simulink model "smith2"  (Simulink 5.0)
settings: Solver=ode45  StartTime=0.0  StopTime=100.0  FixedStep=0.1  RelTol=1e-3
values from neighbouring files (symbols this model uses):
  D = uicontrol(gcf,   'Style','edit',   'ForegroundColor','black',   'BackgroundColor',[1 1 1],   'String',num2str(D),   'Position',[100 18 80 20],   'CallBack',['D=str2num(get(D,''String''));'])    [sus1.m]    (also in sus2.m = uicontrol(gcf,   'Style','edit',   'ForegroundColor','black')
  p0 = P(3,1)    [simulacia11.m]    (also in simulacia12.m = P(1,4); simulacia21.m = P(1,4); simulacia22.m = P(1,5); smith.m = P(2,1))
  p1 = P(2,1)    [simulacia11.m]    (also in simulacia12.m = P(1,3); simulacia21.m = P(1,3); simulacia22.m = P(1,4); smith.m = P(1,1))
  p2 = P(1,1)    [simulacia11.m]    (also in simulacia12.m = P(1,2); simulacia21.m = P(1,2); simulacia22.m = P(1,3); smith.m = 0)
  p3 = 0    [simulacia11.m]    (also in simulacia12.m = P(1,1); simulacia21.m = P(1,1); simulacia22.m = P(1,2); smith.m)
  p4 = 0    [simulacia21.m]    (also in simulacia22.m = P(1,1); smithd.m)
  q0 = P(6,1)    [simulacia11.m]    (also in simulacia12.m = Q(1,4); simulacia21.m = Q(1,4); simulacia22.m = Q(1,5); smith.m = P(4,1))
  q1 = P(5,1)    [simulacia11.m]    (also in simulacia12.m = Q(1,3); simulacia21.m = Q(1,3); simulacia22.m = Q(1,4); smith.m = P(3,1))
  q2 = P(4,1)    [simulacia11.m]    (also in simulacia12.m = Q(1,2); simulacia21.m = Q(1,2); simulacia22.m = Q(1,3); smith.m = 0)
  q3 = 0    [simulacia11.m]    (also in simulacia12.m = Q(1,1); simulacia21.m = Q(1,1); simulacia22.m = Q(1,2); smith.m)
  q4 = 0    [simulacia21.m]    (also in simulacia22.m = Q(1,1); smithd.m)
  T = uicontrol(gcf,   'Style','edit',   'ForegroundColor','black',   'BackgroundColor',[1 1 1],   'String',num2str(T),   'Position',[100 40 80 20],   'CallBack',['T=str2num(get(T,''String''));'])    [sus1.m]    (also in sus2.m = uicontrol(gcf,   'Style','edit',   'ForegroundColor','black')
  Xi = uicontrol(gcf,   'Style','edit',   'ForegroundColor','black',   'BackgroundColor',[1 1 1],   'String',num2str(Xi),   'Position',[100 75 80 20],   'CallBack',['Xi=str2num(get(Xi,''String''));'])    [sus2.m]
  Z = uicontrol(gcf,   'Style','edit',   'ForegroundColor','black',   'BackgroundColor',[1 1 1],   'String',num2str(Z),   'Position',[100 62 80 20],   'CallBack',['Z=str2num(get(Z,''String''));'])    [sus1.m]    (also in sus2.m = uicontrol(gcf,   'Style','edit',   'ForegroundColor','black')

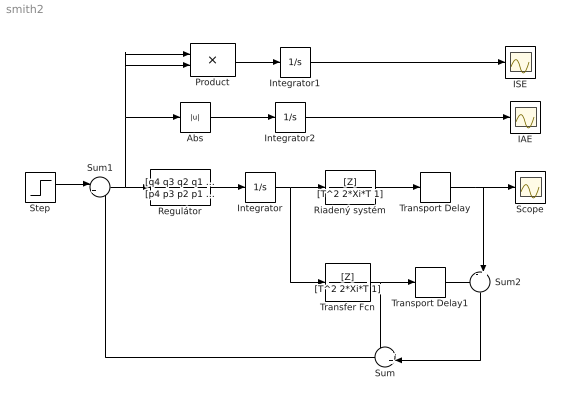
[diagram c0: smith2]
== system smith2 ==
  Abs : Abs
  IAE : Scope
  ISE : Scope
  Integrator : Integrator
  Integrator1 : Integrator
  Integrator2 : Integrator
  Product : Product
  Regulátor : TransferFcn  Numerator=[q4 q3 q2 q1 q0]  Denominator=[p4 p3 p2 p1 p0]
  Riadený systém : TransferFcn  Numerator=[Z]  Denominator=[T^2 2*Xi*T 1]
  Scope : Scope
  Step : Step  SampleTime=0
  Sum : Sum  Orientation=left  Inputs=++|
  Sum1 : Sum  Inputs=|+-
  Sum2 : Sum  Orientation=down  Inputs=-+|
  Transfer Fcn : TransferFcn  Numerator=[Z]  Denominator=[T^2 2*Xi*T 1]
  Transport Delay : TransportDelay  DelayTime=D
  Transport Delay1 : TransportDelay  DelayTime=D
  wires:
  Step/1 -> Sum1/1
  Sum1/1 -> Regulátor/1, Abs/1, Product/1, Product/2
  Regulátor/1 -> Integrator/1
  Integrator/1 -> Riadený systém/1, Transfer Fcn/1
  Riadený systém/1 -> Transport Delay/1
  Transport Delay/1 -> Scope/1, Sum2/2
  Abs/1 -> Integrator2/1
  Integrator2/1 -> IAE/1
  Product/1 -> Integrator1/1
  Integrator1/1 -> ISE/1
  Transfer Fcn/1 -> Transport Delay1/1, Sum/1
  Transport Delay1/1 -> Sum2/1
  Sum2/1 -> Sum/2
  Sum/1 -> Sum1/2
